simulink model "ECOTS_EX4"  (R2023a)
settings: Solver=ode23tb  StartTime=0.0  StopTime=meas.Time(end)  RelTol=1e-3
undefined symbols (not defined in the file or in its folder): mm
libraries: component_lib x15, slpidlib x1

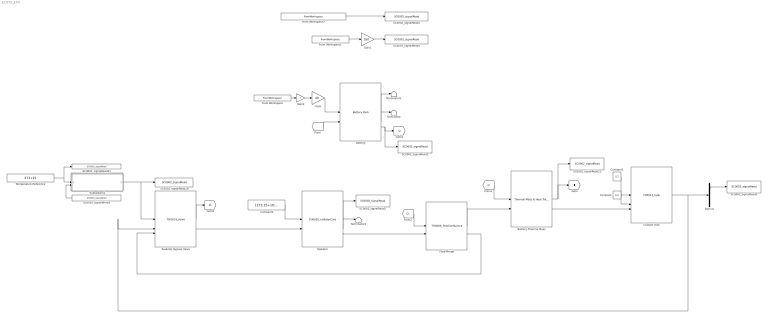
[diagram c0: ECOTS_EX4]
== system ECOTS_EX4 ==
  Battery : component_lib/Battery Pack  SOC_0=1  Nx=40  Ny=180
  Battery Thermal Mass : component_lib/Thermal Mass & Heat Transfer  n=100  d=10e-3  L=4  m=40 * 180 * 0.048  cp=1040  T_0=273 + 25
  Constant : Constant  Value=2e5
  Constant1 : Constant  Value=0.2
  Constant2 : Constant  Value=[273.15+10; 1e5; 5]
  Coolant Tank : component_lib/Thermal Systems/TH0013_tank  V=5e-3  T0=273.15 + 25
  Demux : Demux  Outputs=3
  Flow Merge : component_lib/Thermal Systems/TH0006_flowConfluence  gain=0.01
  From Workspace : FromWorkspace  VariableName=[meas.Time, meas.Current]
  From Workspace1 : FromWorkspace  VariableName=[meas.Time, meas.Voltage]
  From Workspace2 : FromWorkspace  VariableName=[meas.Time, meas.Battery_Temp_degC + 273.15]
  Gain : Gain  Gain=40
  Gain1 : Gain  Gain=180
  Gain2 : Gain  Gain=-1
  Radiator : component_lib/Thermal Systems/TH0002_radiatorCore  HtH=1.1  StS=0.95  radmodel=52 mm
  Radiator Bypass Valve : component_lib/Thermal Systems/TH0014_valve  d=10e-2  dr=5e-2  C_d=0.9
  SC0002_signalRead1 : component_lib/Data & Control/SC0002_signalRead  SigName=generatedHeat
  SC0002_signalRead19 : component_lib/Data & Control/SC0002_signalRead  SigName=radiatorBypassValve
  SC0002_signalRead2 : component_lib/Data & Control/SC0002_signalRead  SigName=radiatorCooling
  SC0002_signalRead21 : component_lib/Data & Control/SC0002_signalRead  SigName=batteryTemperatureReference
  SC0002_signalRead22 : component_lib/Data & Control/SC0002_signalRead  SigName=batteryTemperature
  SC0002_signalRead3 : component_lib/Data & Control/SC0002_signalRead  SigName=coolantTemperature
  SC0002_signalRead4 : component_lib/Data & Control/SC0002_signalRead  SigName=measuredBatteryVoltage
  SC0002_signalRead5 : component_lib/Data & Control/SC0002_signalRead  SigName=measuredBatteryTemperature
  SC0003_signalWrite3 : component_lib/Data & Control/SC0003_signalWrite  SigName=batteryTemperature
  Subsystem1 : Subsystem
  Temperature Reference : Constant  Value=273+25
  Terminator : Terminator
  Terminator1 : Terminator
  Terminator2 : Terminator
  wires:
  Battery/2 -> Terminator/1
  Battery/1 -> Terminator1/1
  Battery Thermal Mass/2 -> Coolant Tank/3
  Battery Thermal Mass/1 -> [T], SC0002_signalRead22/1
  [T] -> Battery/2
  Battery/3 -> SC0002_signalRead1/1, [Q]
  [Q] -> Battery Thermal Mass/1
  Constant/1 -> Coolant Tank/2
  Constant1/1 -> Coolant Tank/1
  Coolant Tank/1 -> Radiator Bypass Valve/2, Demux/1
  Constant2/1 -> Radiator/1
  Radiator/2 -> Terminator2/1
  Radiator/1 -> SC0002_signalRead2/1
  Demux/1 -> SC0002_signalRead3/1
  Flow Merge/1 -> Battery Thermal Mass/2
  Flow Merge/2 -> Radiator Bypass Valve/3
  Subsystem1/1(cv [-]) -> Radiator Bypass Valve/1, SC0002_signalRead19/1
  Temperature Reference/1 -> SC0002_signalRead21/1, Subsystem1/1(T_ref [K])
  SC0003_signalWrite3/1 -> Subsystem1/2(T_fc [K])
  Radiator Bypass Valve/2 -> Radiator/2
  Radiator Bypass Valve/1 -> [CL]
  [CL] -> Flow Merge/1
  Radiator/3 -> Flow Merge/2
  From Workspace2/1 -> SC0002_signalRead5/1
  From Workspace1/1 -> Gain1/1
  Gain1/1 -> SC0002_signalRead4/1
  From Workspace/1 -> Gain2/1
  Gain2/1 -> Gain/1
  Gain/1 -> Battery/1

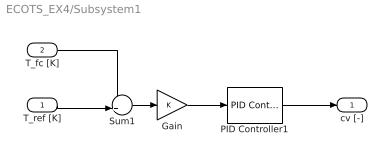
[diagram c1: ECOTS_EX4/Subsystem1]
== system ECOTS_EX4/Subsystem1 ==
  T_ref [K] : Inport
  T_fc [K] : Inport  Port=2
  Gain : Gain
  PID Controller1 : slpidlib/PID Controller  Controller=PI  Form=Parallel  TimeDomain=Continuous-time  UseExternalTs=off  SampleTime=-1  IntegratorMethod=Forward Euler  FilterMethod=Forward Euler  ControllerParametersSource=internal  P=0.2  I=1e-3  UseKiTs=off  D=0  N=100  UseFilter=on  TunerSelectOption=Transfer Function Based (PID Tuner App)  ZeroCross=off  InitialConditionSource=internal  InitialConditionForIntegrator=0.5  InitialConditionForFilter=0.5  DifferentiatorICPrevScaledInput=0  ExternalReset=none  TrackingMode=off  Kt=1  LimitOutput=on  SatLimitsSource=internal  UpperSaturationLimit=1  LowerSaturationLimit=0  LinearizeAsGain=on  AntiWindupMode=clamping  Kb=1  LimitIntegrator=off  UpperIntegratorSaturationLimit=inf  LowerIntegratorSaturationLimit=-inf  POutMin=[]  POutMax=[]  IOutMin=[]  IOutMax=[]  DOutMin=[]  DOutMax=[]  NOutMin=[]  NOutMax=[]  SumOutMin=[]  SumOutMax=[]  SaturationOutMin=[]  SaturationOutMax=[]  PParamMin=[]  PParamMax=[]  IParamMin=[]  IParamMax=[]  DParamMin=[]  DParamMax=[]  NParamMin=[]  NParamMax=[]  KbParamMin=[]  KbParamMax=[]  KtParamMin=[]  KtParamMax=[]  KbOutMin=[]  KbOutMax=[]  KtOutMin=[]  KtOutMax=[]  IntegratorOutMin=[]  IntegratorOutMax=[]  FilterOutMin=[]  FilterOutMax=[]  SumI1OutMin=[]  SumI1OutMax=[]  SumI2OutMin=[]  SumI2OutMax=[]  SumI3OutMin=[]  SumI3OutMax=[]  SumI4OutMin=[]  SumI4OutMax=[]  SumDOutMin=[]  SumDOutMax=[]  DifferentiatorOutMin=[]  DifferentiatorOutMax=[]  FilterDiffOutCoefMin=[]  FilterDiffOutCoefMax=[]  ReciprocalOutMin=[]  ReciprocalOutMax=[]  SumDenOutMin=[]  SumDenOutMax=[]  SumNumOutMin=[]  SumNumOutMax=[]  DivideOutMin=[]  DivideOutMax=[]  UdiffTsProdOutMin=[]  UdiffTsProdOutMax=[]  NTsProdOutMin=[]  NTsProdOutMax=[]  UintegralTsProdOutMin=[]  UintegralTsProdOutMax=[]  UngainTsProdOutMin=[]  UngainTsProdOutMax=[]  ClampingZeroOutDataTypeStr=Inherit: Inherit via back propagation  ClampingZeroOutMin=[]  ClampingZeroOutMax=[]  FilterDenConstantOutDataTypeStr=Inherit: Inherit via back propagation  FilterDenConstantOutMin=[]  FilterDenConstantOutMax=[]  PCopyOutDataTypeStr=Inherit: Inherit via back propagation  PCopyOutMin=[]  PCopyOutMax=[]  NCopyOutDataTypeStr=Inherit: Inherit via back propagation  NCopyOutMin=[]  NCopyOutMax=[]  IntegratorContinuousStateAttributes=''  IntegratorStateMustResolveToSignalObject=off  IntegratorRTWStateStorageClass=Auto  FilterContinuousStateAttributes=''  FilterStateMustResolveToSignalObject=off  FilterRTWStateStorageClass=Auto  ParallelPVariant=InternalParameters  IdealPVariant=Disabled  IVariant=InternalParameters  DVariant=Disabled  IntegratorVariant=Continuous  SatVariant=Enabled  AWVariant=ContClampingParallel  PCopyVariant=Disabled  TRVariant=Disabled  FdbkBlocksVariant=Forward  IdealPFdbkVariant=Disabled  SatFdbkVariant=Disabled  DerivativeFilterVariant=Disabled  NVariant=Disabled  NCopyVariant=Disabled_SignalSpec  FilterICVariant=Disabled  IntegratorICVariant=InternalICs  ExternalResetVariant=Disabled  TRSumVariant=Passthrough  SumFdbkVariant=Disabled  SumVariant=Sum_PI  TsampFilterVariant=InternalTs  TsampNgainVariant=Passthrough  TsampIntegralVariant=Disabled_SignalSpec  ExternalSaturationOutDataTypeStr=Inherit: Same as second input
  Sum1 : Sum  Inputs=-+|
  cv [-] : Outport
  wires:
  T_fc [K]/1 -> Sum1/1
  Gain/1 -> PID Controller1/1
  Sum1/1 -> Gain/1
  PID Controller1/1 -> cv [-]/1
  T_ref [K]/1 -> Sum1/2
